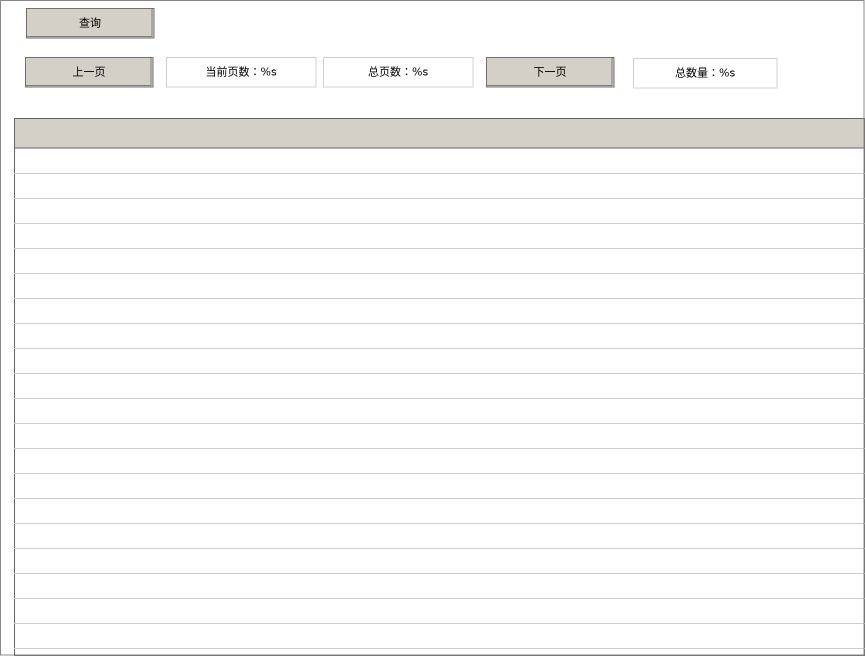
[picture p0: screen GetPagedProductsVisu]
VISUALIZATION GetPagedProductsVisu  // 865x656
    Table (14,118 851x538), data array: MAIN.fbGetPagedProducts.products
        p338671338: MAIN.fbGetPagedProducts.products[INDEX].BarCode
        p2170511999: MAIN.fbGetPagedProducts.products[INDEX].FinalPressure
        p3723444502: MAIN.fbGetPagedProducts.products[INDEX].FinalDisplacement
        p1218418051: MAIN.fbGetPagedProducts.products[INDEX].IsQualified
        p511219082: CreatDateTime
        p1892666644: MAIN.fbGetPagedProducts.products[INDEX].CreatDateTime
        p3854506369: MAIN.fbGetPagedProducts.products[INDEX].Id
    Button (25,57 128x30), "上一页"
        tap MAIN.fbGetPagedProducts.bPreviousPage
    Textfield (166,57 150x30), "当前页数：%s", text variable: MAIN.fbGetPagedProducts.nCurrentPage
    Textfield (323,57 150x30), "总页数：%s", text variable: MAIN.fbGetPagedProducts.nTotalPages
    Button (486,57 128x30), "下一页"
        tap MAIN.fbGetPagedProducts.bNextPage
    Textfield (633,58 144x30), "总数量：%s", text variable: MAIN.fbGetPagedProducts.nTotalItems
    Button (26,8 128x30), "查询"
        tap MAIN.fbGetPagedProducts.bSearch
END_VISUALIZATION
